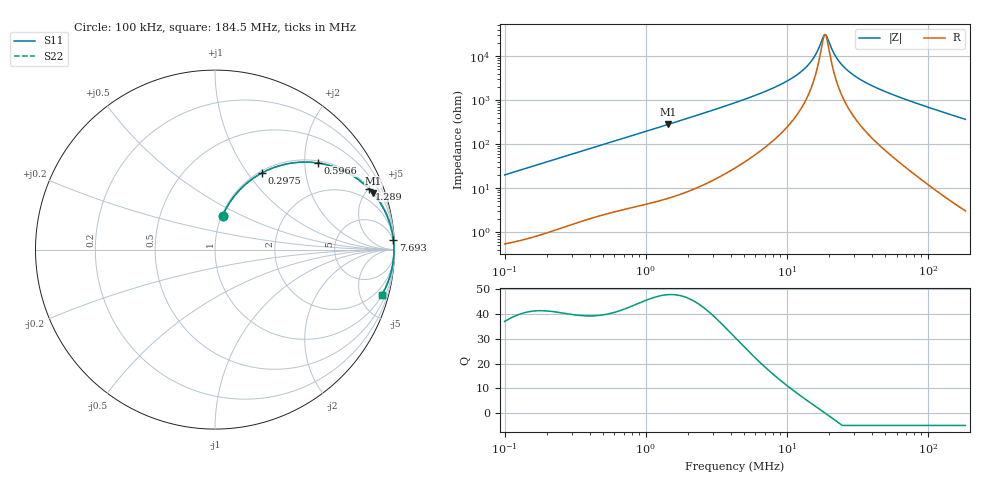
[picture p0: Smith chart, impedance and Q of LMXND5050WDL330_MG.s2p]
! LMXND5050WDL330_MG  S-PARAMETER MODEL  ( General Type )
! Model Generated by TAIYO YUDEN Corporation (http://www.ty-top.com)
! Version 1.0
! TAIYO YUDEN Control No. 191023NI43SB-FBB
! Copyright(c) 2019 TAIYO YUDEN CO.,LTD. All Rights Reserved.
! Product Description (link to TY-COMPAS)
! https://ds.yuden.co.jp/TYCOMPAS/or/detail?pn=LMXND5050WDL330MMG&u=M
! Products Name : Inductors
! Characteristics :
!  Inductance : 33 uH , SRF(min) : 11 MHz , DC Resistance(max) : 0.444 Ohm
!  Rated Current : Saturation :1000 mA , Temp Rise : 630 mA
!  Case Size : 4.9 x 4.9 / 0.193 x 0.193 [mm/inch] , Thickness : 2.4 / 0.094 [mm/inch]
!  (Conditions: Temperature = 25 degC , DC Bias Current/Voltage = 0A / 0V)
! External Node Assignments :
!  1  o---GGG---o  2
! GND o---------o GND
! Frequency Range : 0.1MHz  -  184.468258MHz  [ 402 STEP ]
# MHz S RI R 50
! Freq[MHz].  S11 Real  S11 Imag  S21 Real  S21 Imag  S12 Real  S12 Imag  S22 Real  S22 Imag
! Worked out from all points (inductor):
!   401 points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, 100 kHz to 184.5 MHz, reference 50 ohm
!   read as one part in series: L = 31.6 uH near 103.8 kHz
!   highest Q = 47.8 at 1.443 MHz (marker M1), where L = 30.8 uH
!   self-resonance near 18.61 MHz
!   S11 on the Smith chart (normalised r, x): 100 kHz: 1.01, +0.40; 297.5 kHz: 1.03, +1.17; 596.6 kHz: 1.06, +2.32; 1.289 MHz: 1.11, +4.99; 7.693 MHz: 3, +35; 184.5 MHz: 1.06, -7.28
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0.1  0.0428 0.1893  0.9572 -0.1893  0.9572 -0.1893  0.0428 0.1893
0.179106  0.1178 0.3105  0.8822 -0.3105  0.8822 -0.3105  0.1178 0.3105
0.297549  0.261 0.4268  0.739 -0.4268  0.739 -0.4268  0.261 0.4268
0.352405  0.3282 0.457  0.6718 -0.457  0.6718 -0.457  0.3282 0.457
0.596563  0.5727 0.4825  0.4273 -0.4825  0.4273 -0.4825  0.5727 0.4825
1.241892  0.8474 0.3492  0.1526 -0.3492  0.1526 -0.3492  0.8474 0.3492
1.289476  0.8566 0.3401  0.1434 -0.3401  0.1434 -0.3401  0.8566 0.3401
1.443451  0.8816 0.3128  0.1184 -0.3128  0.1184 -0.3128  0.8816 0.3128
4.294977  0.9834 0.1125  0.0166 -0.1125  0.0166 -0.1125  0.9834 0.1125
7.69254  0.9935 0.0557  0.00651 -0.0557  0.00651 -0.0557  0.9935 0.0557
11.6331  0.996 0.0272  0.00403 -0.0272  0.00403 -0.0272  0.996 0.0272
13.52116  0.9964 0.0182  0.00359 -0.0182  0.00359 -0.0182  0.9964 0.0182
15.13571  0.9966 0.0117  0.00338 -0.0117  0.00338 -0.0117  0.9966 0.0117
16.31781  0.9967 0.00752  0.00329 -0.00752  0.00329 -0.00752  0.9967 0.00752
17.9261  0.9968 0.00229  0.00322 -0.00229  0.00322 -0.00229  0.9968 0.00229
18.61296  0.9968 0.000203  0.00321 -0.000203  0.00321 -0.000203  0.9968 0.000203
18.9662  0.9968 -0.000839  0.00321 0.000839  0.00321 0.000839  0.9968 -0.000839
22.46278  0.9967 -0.0103  0.00329 0.0103  0.00329 0.0103  0.9967 -0.0103
26.60399  0.9965 -0.02  0.00355 0.02  0.00355 0.02  0.9965 -0.02
35.27109  0.9955 -0.0376  0.00449 0.0376  0.00449 0.0376  0.9955 -0.0376
53.33896  0.9923 -0.0693  0.00773 0.0693  0.00773 0.0693  0.9923 -0.0693
184.4683  0.928 -0.2543  0.072 0.2543  0.072 0.2543  0.928 -0.2543
